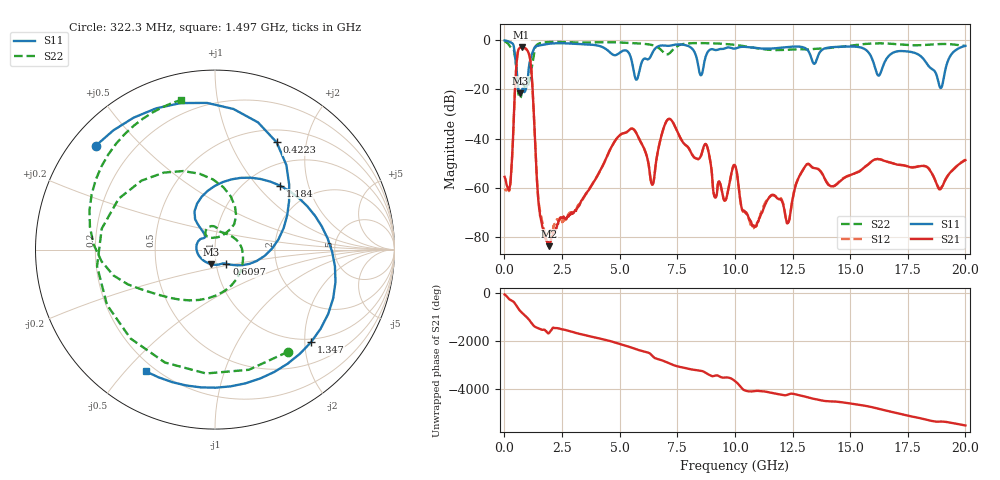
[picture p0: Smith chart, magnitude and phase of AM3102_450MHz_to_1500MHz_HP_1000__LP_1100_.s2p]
!Agilent Technologies,E8364B,MY43040894,A.07.50.67
!Agilent E8364B: A.07.50.67
!Date: Thursday, January 11, 2018 05:59:34
!Correction: S11(Full 2 Port(1,2))
!S21(Full 2 Port(1,2))
!S12(Full 2 Port(1,2))
!S22(Full 2 Port(1,2))
!S2P File: Measurements: S11, S21, S12, S22:
# Hz S  dB  R 50
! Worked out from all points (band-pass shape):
!   1601 points, 10 MHz to 20 GHz, reference 50 ohm
!   highest |S21| = -2.92 dB at 747.1 MHz (marker M1); lowest = -83.8 dB at 1.934 GHz (marker M2)
!   |S21| within 3 dB of the highest: 566.1 MHz to 1.079 GHz (513 MHz wide, 62.4 % of centre)
!   lowest |S11| = -21.5 dB at 697.2 MHz (marker M3), VSWR 1.18, Z = 47.2 - j7.69 ohm
!   |S11| at or under -10 dB: 510.2 MHz to 1.078 GHz (567.9 MHz wide, 71.5 % of centre); 16.05 GHz to 16.45 GHz (402 MHz wide, 2.47 % of centre); 18.36 GHz to 19.18 GHz (820.2 MHz wide, 4.37 % of centre)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
!   |S22| runs from -23.5 to -0.5 dB; largest |S21 - S12| = 0.00084
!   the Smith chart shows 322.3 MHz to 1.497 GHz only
!   S11 on the Smith chart (normalised r, x): 322.3 MHz: 0.07, +0.37; 422.3 MHz: 0.67, +1.52; 609.7 MHz: 1.12, -0.18; 1.184 GHz: 1.39, +1.34; 1.347 GHz: 0.93, -2.14; 1.497 GHz: 0.16, -0.57
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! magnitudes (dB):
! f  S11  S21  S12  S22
! 10 MHz  -0.1  -55.6  -60.5  -0.5
! 322.3 MHz  -1.1  -49.6  -49.9  -3.1
! 422.3 MHz  -3.2  -28.2  -28.2  -4.3
! 609.7 MHz  -19.9  -3.8  -3.8  -22.0
! 697.2 MHz  -21.5  -3.0  -3.0  -23.4
! 747.1 MHz  -20.8  -2.9  -2.9  -21.5
! 1.184 GHz  -5.9  -14.1  -14.1  -11.3
! 1.347 GHz  -2.6  -44.8  -44.8  -2.7
! 1.497 GHz  -2.2  -67.4  -66.6  -1.4
! 1.934 GHz  -1.4  -83.8  -78.4  -0.7
! 3.346 GHz  -1.6  -65.2  -65.6  -1.0
! 5.045 GHz  -4.8  -38.3  -38.4  -0.9
! 6.407 GHz  -5.4  -58.7  -58.8  -1.9
! 6.682 GHz  -2.4  -44.1  -44.1  -3.0
! 8.743 GHz  -6.4  -42.3  -42.3  -1.2
! 9.568 GHz  -3.3  -65.2  -65.1  -1.5
! 10.01 GHz  -3.4  -51.0  -51.0  -1.9
! 10.82 GHz  -3.1  -75.3  -76.4  -3.0
! 13.34 GHz  -8.0  -51.6  -51.6  -3.6
! 16.68 GHz  -6.3  -49.6  -49.6  -1.4
! 18.93 GHz  -19.4  -60.6  -60.2  -1.5
! 20 GHz  -2.3  -48.8  -48.6  -2.3
